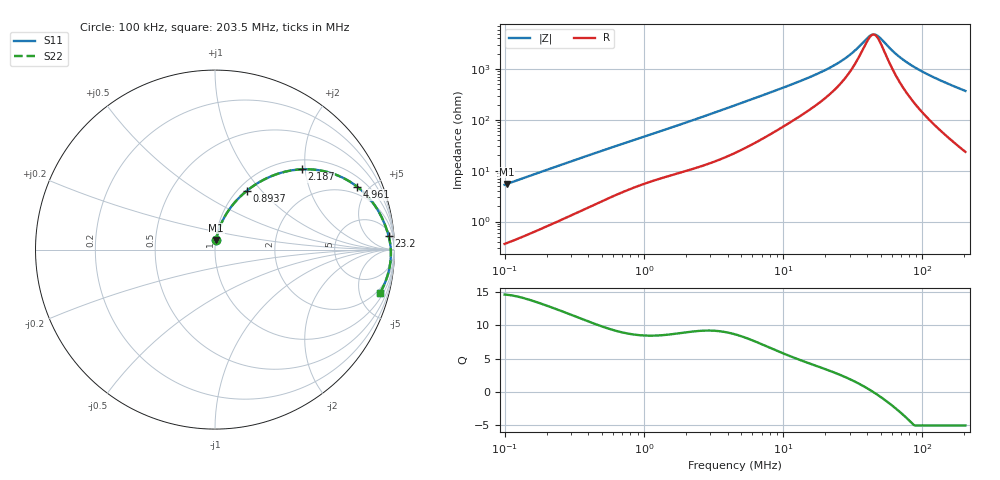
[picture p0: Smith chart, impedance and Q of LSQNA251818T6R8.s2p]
! LSQNA251818T6R8  S-PARAMETER MODEL  ( General Type )
! Model Generated by TAIYO YUDEN Corporation (http://www.ty-top.com)
! Version 2.0
! TAIYO YUDEN Control No. 100810NF25SB-FKC
! Copyright(c) 2007 TAIYO YUDEN CO.,LTD. All Rights Reserved.
! Product Description (link to TY-COMPAS)
! https://ds.yuden.co.jp/TYCOMPAS/or/detail?pn=LSQNA251818T6R8M&u=M
! Products Name : Inductors
! Characteristics :
!  Inductance : 6.8 uH , SRF(min) : 38 MHz , DC Resistance(max) : 0.195 Ohm
!  Rated Current : Saturation :270 mA , Temp Rise : 930 mA (40 degC)
!  Case Size : 2.5 x 1.8 / 0.098 x 0.071 [mm/inch] , Thickness : 1.8 / 0.071 [mm/inch]
!  (Conditions: Temperature = 25 degC , DC Bias Current/Voltage = 0A / 0V)
! External Node Assignments :
!  1  o---GGG---o  2
! GND o---------o GND
! Frequency Range : 0.1MHz  -  203.457813MHz  [ 402 STEP ]
# MHz S RI R 50
! Freq[MHz].  S11 Real  S11 Imag  S21 Real  S21 Imag  S12 Real  S12 Imag  S22 Real  S22 Imag
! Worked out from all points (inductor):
!   401 points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, 100 kHz to 203.5 MHz, reference 50 ohm
!   read as one part in series: L = 8.35 uH near 103.9 kHz
!   highest Q = 14.5 at 103.9 kHz (marker M1), where L = 8.4 uH
!   self-resonance near 44.32 MHz
!   S11 on the Smith chart (normalised r, x): 100 kHz: 1.01, +0.11; 893.7 kHz: 1.10, +0.84; 2.187 MHz: 1.21, +1.91; 4.961 MHz: 1.51, +4.23; 23.2 MHz: 9, +22; 203.5 MHz: 1.47, -7.41
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0.1  0.00637 0.0523  0.9936 -0.0523  0.9936 -0.0523  0.00637 0.0523
0.103882  0.00672 0.0542  0.9933 -0.0542  0.9933 -0.0542  0.00672 0.0542
0.358236  0.0461 0.1689  0.9539 -0.1689  0.9539 -0.1689  0.0461 0.1689
0.576699  0.0962 0.2463  0.9038 -0.2463  0.9038 -0.2463  0.0962 0.2463
0.893689  0.1778 0.3282  0.8222 -0.3282  0.8222 -0.3282  0.1778 0.3282
1.283332  0.2783 0.3929  0.7217 -0.3929  0.7217 -0.3929  0.2783 0.3929
2.18742  0.4825 0.4473  0.5175 -0.4473  0.5175 -0.4473  0.4825 0.4473
3.081864  0.6276 0.432  0.3724 -0.432  0.3724 -0.432  0.6276 0.432
4.51063  0.7648 0.3701  0.2352 -0.3701  0.2352 -0.3701  0.7648 0.3701
4.961273  0.7924 0.3501  0.2076 -0.3501  0.2076 -0.3501  0.7924 0.3501
8.296886  0.8953 0.2386  0.1047 -0.2386  0.1047 -0.2386  0.8953 0.2386
16.15871  0.9526 0.1233  0.0474 -0.1233  0.0474 -0.1233  0.9526 0.1233
23.2038  0.9674 0.0754  0.0326 -0.0754  0.0326 -0.0754  0.9674 0.0754
30.29394  0.9744 0.0436  0.0256 -0.0436  0.0256 -0.0436  0.9744 0.0436
40.311  0.9788 0.0109  0.0212 -0.0109  0.0212 -0.0109  0.9788 0.0109
43.50191  0.9794 0.00214  0.0206 -0.00214  0.0206 -0.00214  0.9794 0.00214
47.84805  0.98 -0.00887  0.02 0.00887  0.02 0.00887  0.98 -0.00887
57.88634  0.9801 -0.0315  0.0199 0.0315  0.0199 0.0315  0.9801 -0.0315
71.37714  0.9784 -0.0579  0.0216 0.0579  0.0216 0.0579  0.9784 -0.0579
93.18709  0.9732 -0.0951  0.0268 0.0951  0.0268 0.0951  0.9732 -0.0951
133.8161  0.9579 -0.1553  0.0421 0.1553  0.0421 0.1553  0.9579 -0.1553
203.4578  0.9191 -0.2429  0.0809 0.2429  0.0809 0.2429  0.9191 -0.2429
